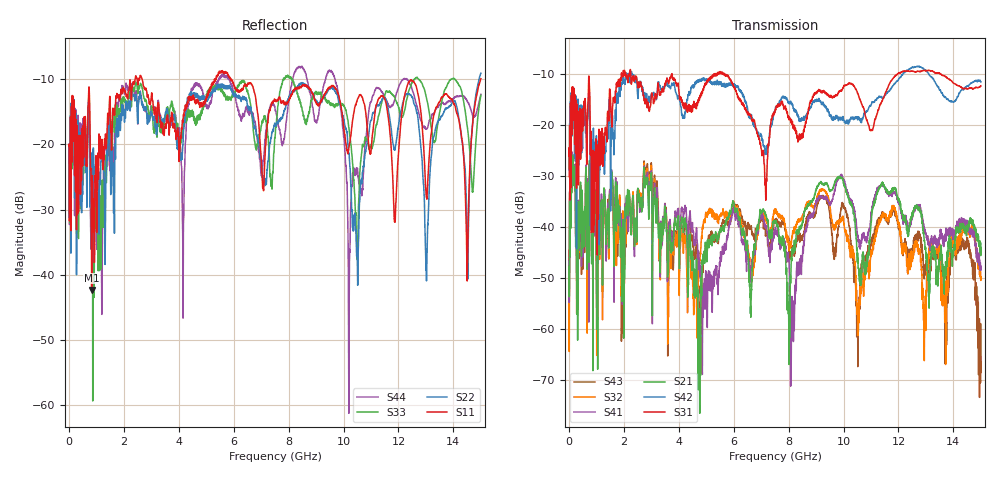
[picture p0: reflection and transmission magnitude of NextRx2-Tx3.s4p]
! FILE: N:\QM 2007\Prüfprotokolle\Highspeed\Konfektionierte Ltg\L45593-D106\D30\8216\0002\Next  Platine 2\NextRx2-Tx3.s4p
# MHz S DB R 50.00
! FREQ  S11  S12  S13  S14
!  S21  S22  S23  S24
!  S31  S32  S33  S34
!  S41  S42  S43  S44
!  DB  ANG  DB  ANG  DB  ANG  DB  ANG
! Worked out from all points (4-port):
!   2999 points, 10 MHz to 15 GHz, reference 50 ohm
!   strongest paths, dB at 10 MHz, 3.755 GHz, 7.505 GHz, 11.26 GHz, 15 GHz:
!     S31: -26.2, -10.0, -17.3, -17.1, -12.4
!     S42: -25.5, -11.9, -17.5, -14.8, -11.7
!     S21: -47.7, -43.8, -39.0, -33.0, -43.2
!     S41: -46.7, -42.9, -41.3, -32.5, -47.6
!     S32: -46.4, -43.4, -36.5, -39.7, -49.7
!     S43: -44.5, -41.2, -38.9, -39.2, -66.4
!   lowest |S11| = -42.3 dB at 830 MHz (marker M1), VSWR 1.02, Z = 50.7 - j0.229 ohm
!   |S11| at or under -10 dB: start of sweep to 2.415 GHz; 2.664 GHz to 5.332 GHz (2.668 GHz wide, 66.7 % of centre); 5.89 GHz to 15 GHz (9.106 GHz wide, 87.2 % of centre)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
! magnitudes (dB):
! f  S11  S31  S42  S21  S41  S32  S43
! 10 MHz  -20.2  -26.2  -25.5  -47.7  -46.7  -46.4  -44.5
! 830 MHz  -42.3  -31.3  -34.3  -47.2  -45.8  -45.8  -44.7
! 9.515 GHz  -11.3  -14.6  -18.3  -32.8  -35.3  -36.4  -38.3
! 10.21 GHz  -20.1  -11.9  -19.2  -35.0  -34.8  -44.0  -39.8
! 12.38 GHz  -10.5  -9.5  -9.2  -40.4  -40.8  -47.0  -44.4
! 13.02 GHz  -28.1  -9.4  -9.6  -47.0  -42.1  -52.7  -49.3
! 15 GHz  -10.0  -12.4  -11.7  -43.2  -47.6  -49.7  -66.4
